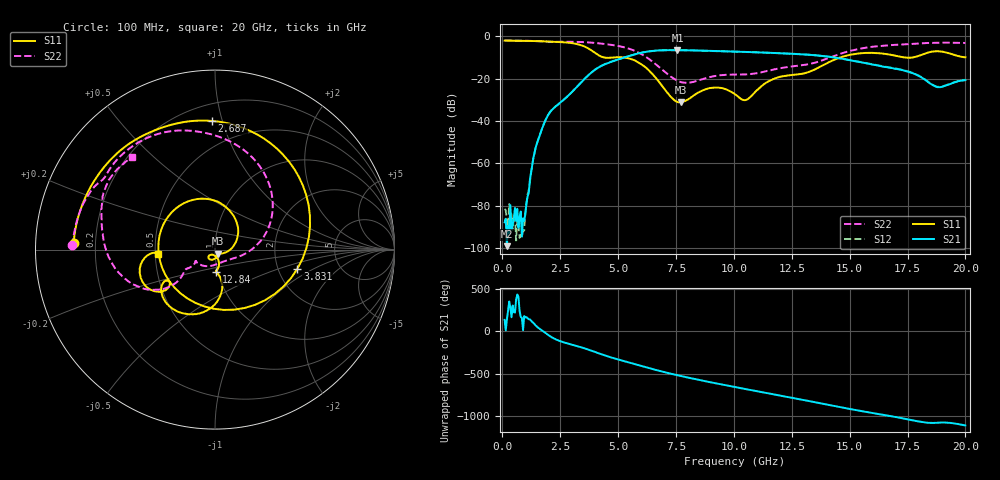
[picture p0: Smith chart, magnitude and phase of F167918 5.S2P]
!  2-Port S-parameters saved by WinCal
! VAR MeasName=S-Parameters (CALIBRATED_DATA) read from VNA (N5242A)
! VAR MeasDate=2016-11-22 10:25:05
! VAR NAME=F167918 5
! VAR FILENAME=F167918 5.S2P
! VAR DATE=2016-11-22 10:25:05
! VAR PHYS_PORTS=1,2
# Hz S DB R 50
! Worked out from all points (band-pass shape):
!   401 points, 100 MHz to 20 GHz, reference 50 ohm
!   highest |S21| = -6.56 dB at 7.562 GHz (marker M1); lowest = -99.0 dB at 199.5 MHz (marker M2)
!   |S21| within 3 dB of the highest: 5.403 GHz to 14.03 GHz (8.628 GHz wide, 88.8 % of centre)
!   lowest |S11| = -31.2 dB at 7.712 GHz (marker M3), VSWR 1.06, Z = 51.4 - j2.4 ohm
!   |S11| at or under -10 dB: 4.383 GHz to 4.835 GHz (452.2 MHz wide, 9.81 % of centre); 5.228 GHz to 14.61 GHz (9.378 GHz wide, 94.6 % of centre); 17.38 GHz to 17.73 GHz (350.6 MHz wide, 2 % of centre)
!   |S22| runs from -22.0 to -2.0 dB; largest |S21 - S12| = 0.0045
!   S11 on the Smith chart (normalised r, x): 100 MHz: 0.12, +0.02; 2.687 GHz: 0.31, +0.93; 3.831 GHz: 2.56, -0.70; 12.84 GHz: 0.98, -0.25; 20 GHz: 0.52, -0.03
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1e8  -2.07 177.3  -87.76 138.3  -81.47 -160.2  -2.00 178.3
1.995e8  -2.08 174.6  -99.03 144.2  -88.35 -17.3  -2.01 176.7
9.4575e8  -2.20 154.6  -86.94 -176.9  -91.66 -100.9  -2.13 164.7
1.692e9  -2.36 132.1  -44.32 16.1  -44.30 15.0  -2.41 152.4
2.687e9  -2.89 91.3  -29.66 -132.1  -29.67 -132.5  -2.60 137.6
3.43325e9  -4.35 36.2  -21.46 169.7  -21.48 169.6  -2.75 121.8
3.83125e9  -6.53 -13.0  -17.28 133.4  -17.28 133.4  -3.00 111.8
4.22925e9  -9.38 -81.7  -14.27 94.2  -14.24 94.2  -3.42 101.1
4.7765e9  -10.06 -174.9  -11.79 45.3  -11.75 45.0  -4.19 84.7
5.52275e9  -10.64 105.0  -9.16 -12.6  -9.17 -13.0  -6.05 55.5
6.7665e9  -21.53 -0.3  -6.70 -106.9  -6.72 -106.9  -14.53 -3.5
7.5625e9  -31.00 -51.3  -6.56 -160.0  -6.58 -160.1  -20.95 -42.2
7.71175e9  -31.17 -57.5  -6.57 -169.4  -6.59 -169.3  -21.62 -51.7
8.9555e9  -24.47 -107.3  -6.90 118.5  -6.88 118.4  -19.31 -122.9
1.005e10  -27.40 -133.7  -7.24 59.7  -7.26 59.7  -18.12 -148.7
1.13435e10  -22.36 -73.4  -7.72 -7.7  -7.72 -7.4  -16.60 -144.7
1.2836e10  -17.92 -86.6  -8.50 -85.0  -8.47 -84.8  -13.84 -145.7
1.338325e10  -16.24 -79.5  -8.86 -114.3  -8.83 -113.8  -12.82 -142.2
1.457725e10  -10.12 -91.4  -10.46 -178.5  -10.38 -178.2  -8.40 -144.3
1.67165e10  -8.67 -144.3  -14.79 76.9  -14.75 76.7  -4.25 178.2
1.8806e10  -7.07 -159.3  -24.03 -4.3  -23.84 -4.4  -3.03 147.4
2e10  -9.93 -175.4  -20.69 -36.5  -20.58 -36.9  -3.18 131.7
